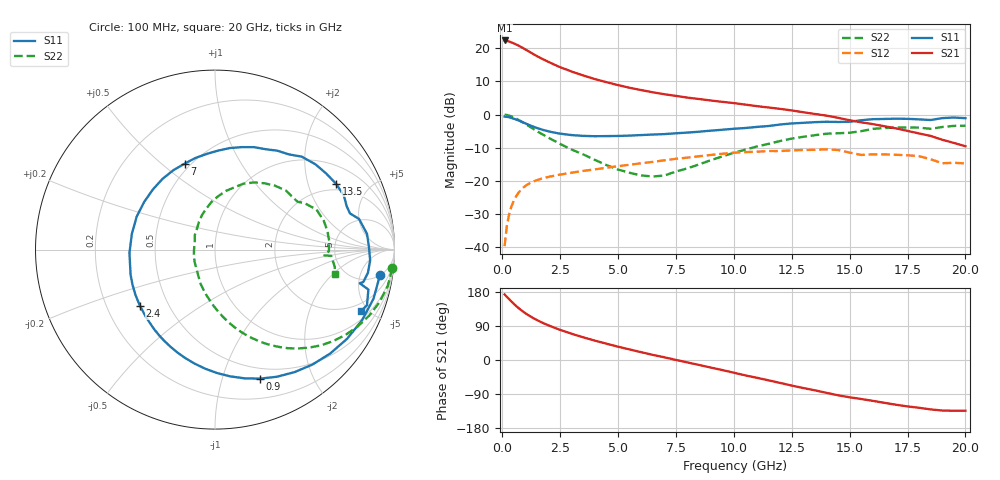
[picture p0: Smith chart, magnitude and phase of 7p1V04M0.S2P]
! Infineon Technologies  Discrete & RF Semiconductors
! bfp620
! VCE =  1.0 V,  IC =  4.0 mA
! Common Emitter S-Parameters:  Sep 2002
# GHz  S  MA  R  50
!  f  S11  S21  S12  S22
! GHz  MAG  ANG  MAG  ANG  MAG  ANG  MAG  ANG
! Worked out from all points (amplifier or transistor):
!   59 points, 100 MHz to 20 GHz, reference 50 ohm
!   highest |S21| = 22.3 dB at 100 MHz (marker M1)
!   |S21| within 3 dB of that: start of sweep to 1.069 GHz
!   unconditionally stable (mu >= 1): 5.123 GHz to 11.81 GHz; 14.7 GHz to 15.51 GHz; 17.03 GHz to end of sweep
!   at 1 GHz: K = 0.27, MSG = 20.6 dB, |S12| = -21.5 dB
!   at 5.5 GHz: K = 1.03, MAG = 10.5 dB, |S12| = -15.1 dB
!   at 20 GHz: K = 1.53, MAG = -1.7 dB, |S12| = -14.7 dB
!   S11 on the Smith chart (normalised r, x): 100 MHz: 5, -11; 900 MHz: 0.39, -1.34; 2.4 GHz: 0.34, -0.30; 7 GHz: 0.46, +0.60; 13.5 GHz: 1.70, +3.05; 20 GHz: 1.44, -4.47
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0.1  0.9304 -8.7  13.07 172.9  0.0104 80.0  0.9934 -6.0
0.2  0.9246 -17.2  12.87 166.5  0.0214 80.5  0.9837 -11.9
0.3  0.9089 -25.7  12.56 160.2  0.0319 76.4  0.9629 -17.6
0.4  0.8881 -34.0  12.2 154.0  0.0417 71.9  0.935 -23.1
0.5  0.8646 -42.0  11.79 148.1  0.0507 67.5  0.9028 -28.4
0.7  0.8139 -57.0  10.92 137.2  0.0664 59.5  0.8316 -37.9
0.9  0.7616 -70.7  10.01 127.7  0.0789 52.8  0.7575 -46.1
1.2  0.6877 -89.1  8.697 115.5  0.0929 44.8  0.6519 -56.4
1.4  0.6457 -100.0  7.927 108.5  0.0998 40.6  0.5897 -62.2
1.6  0.6108 -109.9  7.267 102.2  0.1056 37.1  0.5354 -67.2
2  0.5581 -127.5  6.205 91.3  0.115 31.8  0.447 -75.8
2.4  0.5224 -143.2  5.352 81.7  0.1228 27.7  0.376 -83.4
3  0.4905 -163.6  4.43 69.1  0.1331 22.6  0.2959 -94.0
3.5  0.4769 -177.8  3.875 59.8  0.1416 19.2  0.2505 -102.5
4  0.4715 169.2  3.421 51.1  0.1494 15.9  0.2073 -112.7
5  0.4758 146.0  2.776 35.1  0.1666 9.9  0.1484 -134.0
7  0.5077 109.5  2.023 7.1  0.2042 -2.9  0.1207 159.6
8.5  0.5515 88.3  1.713 -13.1  0.2354 -14.8  0.1774 120.5
10.5  0.6269 63.1  1.411 -40.7  0.2719 -34.7  0.296 87.0
13.5  0.7677 28.6  1.02 -80.0  0.2948 -64.2  0.4887 46.7
17  0.8665 -4.0  0.619 -118.0  0.2475 -94.6  0.6349 9.2
20  0.8818 -23.0  0.333 -133.8  0.1836 -110.2  0.6801 -11.7
